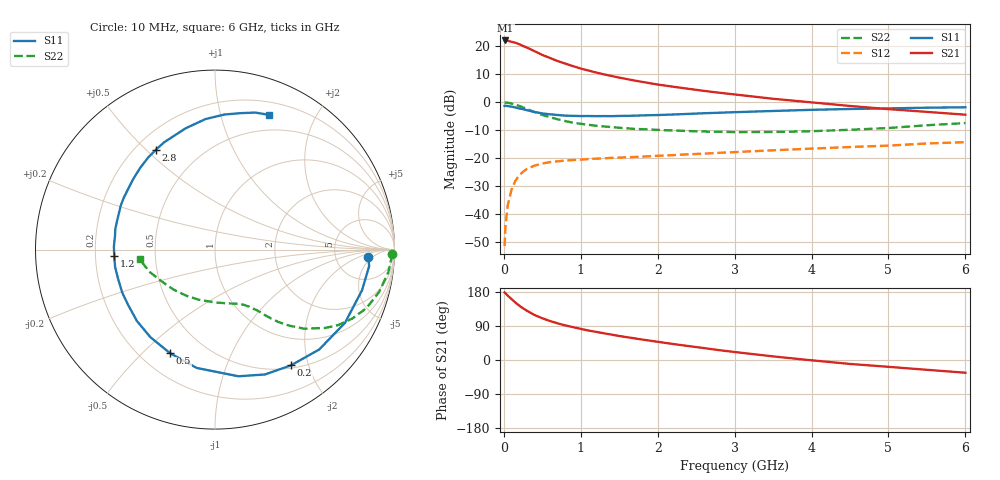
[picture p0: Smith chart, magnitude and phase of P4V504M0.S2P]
! SIEMENS Small Signal Semiconductors
! BFP182
! Si NPN RF Bipolar Junction Transistor in SOT143
! VCE = 0.5 V  IC = 4 mA
! Common Emitter S-Parameters:  March  1996
# GHz  S  MA  R  50
!  f  S11  S21  S12  S22
! GHz  MAG  ANG  MAG  ANG  MAG  ANG  MAG  ANG
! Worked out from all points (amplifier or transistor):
!   36 points, 10 MHz to 6 GHz, reference 50 ohm
!   highest |S21| = 22.0 dB at 20 MHz (marker M1)
!   |S21| within 3 dB of that: start of sweep to 335.9 MHz
!   unconditionally stable (mu >= 1): 1.466 GHz to end of sweep
!   at 250 MHz: K = 0.21, MSG = 22.4 dB, |S12| = -24.8 dB
!   at 1.4 GHz: K = 0.97, MSG = 14.6 dB, |S12| = -19.9 dB
!   at 6 GHz: K = 1.19, MAG = 2.2 dB, |S12| = -14.3 dB
!   S11 on the Smith chart (normalised r, x): 10 MHz: 12, -4; 200 MHz: 0.54, -1.72; 500 MHz: 0.32, -0.61; 1.2 GHz: 0.28, -0.03; 2.8 GHz: 0.28, +0.54; 6 GHz: 0.33, +1.43
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0.01  0.856 -2.9  12.36 178.4  0.0027 86.0  0.9837 -1.4
0.02  0.8638 -6.1  12.58 176.6  0.0059 85.5  0.9837 -3.0
0.05  0.85 -15.4  12.44 170.1  0.0143 84.1  0.974 -7.4
0.1  0.8313 -29.4  11.9 160.8  0.0276 73.4  0.9442 -14.5
0.15  0.8042 -43.8  11.46 151.6  0.0394 65.9  0.9048 -21.1
0.2  0.7715 -56.7  10.79 143.5  0.0497 60.3  0.8556 -26.7
0.25  0.7493 -68.2  10.01 136.3  0.0574 54.4  0.805 -31.5
0.3  0.7178 -79.5  9.404 130.0  0.0644 50.0  0.7549 -35.3
0.4  0.6672 -98.8  8.085 118.6  0.0738 42.3  0.6634 -41.6
0.5  0.6291 -113.4  6.939 110.1  0.0804 36.8  0.592 -45.7
0.6  0.6065 -126.4  6.13 102.9  0.0851 33.1  0.5381 -48.7
0.7  0.5896 -137.5  5.395 96.7  0.088 30.2  0.4937 -50.9
0.8  0.5738 -147.6  4.855 91.2  0.0907 28.1  0.4589 -52.7
1.1  0.5649 -170.1  3.66 77.8  0.0967 24.1  0.3939 -56.9
1.2  0.5627 -176.2  3.375 74.2  0.0981 23.0  0.3792 -58.3
1.7  0.5735 158.5  2.423 57.1  0.1051 21.5  0.3326 -65.0
2.2  0.6015 139.4  1.883 42.2  0.1135 20.5  0.312 -74.2
2.8  0.6471 120.5  1.471 26.0  0.1247 18.9  0.2959 -87.9
3.5  0.6953 103.6  1.148 9.5  0.1383 16.4  0.2934 -107.4
4.5  0.7544 86.0  0.854 -10.4  0.1584 11.8  0.3215 -136.4
5.5  0.7958 73.6  0.67 -25.9  0.183 7.0  0.3869 -161.6
6  0.8093 68.0  0.597 -33.6  0.1932 3.0  0.4232 -172.8
